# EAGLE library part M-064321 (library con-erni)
12 pol. male SMC CONNECTOR vertical , type Q, low profile Source: http://www.erni.com/DB/PDF-Drawing/SMC/064321.pdf
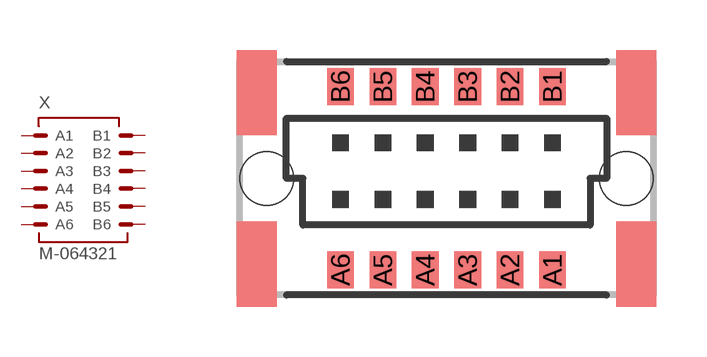
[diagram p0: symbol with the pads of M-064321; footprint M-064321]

Designator prefix X

## M-064321 (OC_FARNELL: unknown; OC_NEWARK: unknown)  [M-064321]
A1  A1  pas
A2  A2  pas
A3  A3  pas
A4  A4  pas
A5  A5  pas
A6  A6  pas
B1  B1  pas
B2  B2  pas
B3  B3  pas
B4  B4  pas
B5  B5  pas
B6  B6  pas

## Footprint M-064321 (pad centres in mm)
12 pol. male SMC CONNECTOR vertical , type Q, low profile Source: http://www.erni.com/DB/PDF-Drawing/SMC/064321.pdf
smd 0.8 x 1.1: A1 3.175,-2.75; A2 1.905,-2.75; A3 0.635,-2.75; A4 -0.635,-2.75; A5 -1.905,-2.75; A6 -3.175,-2.75; B1 3.175,2.75; B2 1.905,2.75; B3 0.635,2.75; B4 -0.635,2.75; B5 -1.905,2.75; B6 -3.175,2.75
hole 1.6 at 5.385,0
hole 1.6 at -5.385,0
